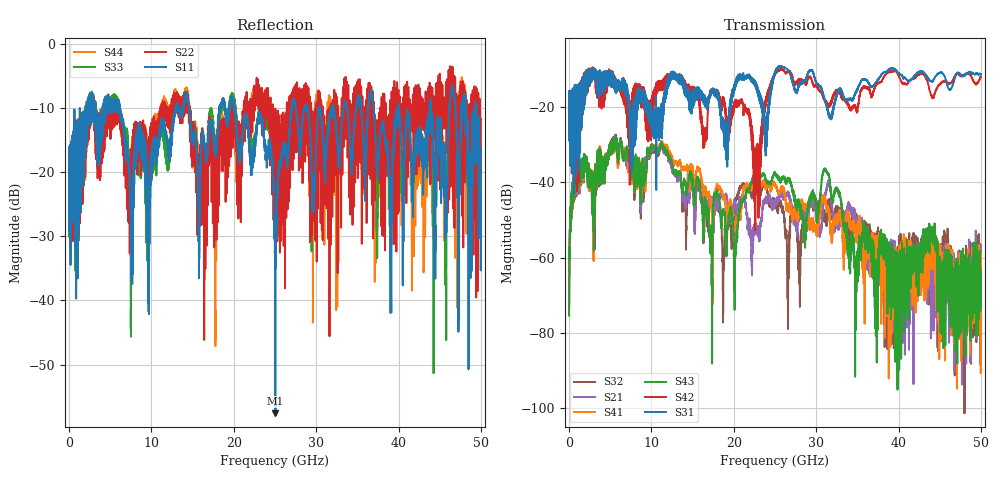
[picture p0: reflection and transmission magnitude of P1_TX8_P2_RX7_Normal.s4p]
!Keysight Technologies,N5225B,MY57041031,A.13.20.10
!Date: Friday, May 31, 2019 11:39:04
!Correction: S11(Full 4 Port(1,2,3,4))
!S12(Full 4 Port(1,2,3,4))
!S13(Full 4 Port(1,2,3,4))
!S14(Full 4 Port(1,2,3,4))
!S21(Full 4 Port(1,2,3,4))
!S22(Full 4 Port(1,2,3,4))
!S23(Full 4 Port(1,2,3,4))
!S24(Full 4 Port(1,2,3,4))
!S31(Full 4 Port(1,2,3,4))
!S32(Full 4 Port(1,2,3,4))
!S33(Full 4 Port(1,2,3,4))
!S34(Full 4 Port(1,2,3,4))
!S41(Full 4 Port(1,2,3,4))
!S42(Full 4 Port(1,2,3,4))
!S43(Full 4 Port(1,2,3,4))
!S44(Full 4 Port(1,2,3,4))
!S4P File: Measurements: <S11,S12,S13,S14>,
!<S21,S22,S23,S24>,
!<S31,S32,S33,S34>,
!<S41,S42,S43,S44>:
# Hz S  dB  R 50.0
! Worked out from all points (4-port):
!   5000 points, 10 MHz to 50 GHz, reference 50 ohm
!   strongest paths, dB at 10 MHz, 12.51 GHz, 25.01 GHz, 37.51 GHz, 50 GHz:
!     S31: -19.6, -10.7, -11.1, -12.7, -11.3
!     S42: -19.3, -12.1, -11.4, -13.7, -12.0
!     S43: -75.4, -35.1, -37.6, -66.2, -70.9
!     S41: -65.5, -33.4, -40.2, -55.2, -60.5
!     S21: -62.9, -36.6, -44.9, -58.5, -62.3
!     S32: -63.7, -36.4, -45.9, -56.3, -66.4
!   lowest |S11| = -57.6 dB at 25.05 GHz (marker M1), VSWR 1.00, Z = 49.9 - j0.0463 ohm
!   |S11| at or under -10 dB: 6.186 GHz to 12.89 GHz (6.703 GHz wide, 70.3 % of centre); 20.1 GHz to 26.99 GHz (6.891 GHz wide, 29.3 % of centre); 40 GHz to 43.77 GHz (3.763 GHz wide, 8.98 % of centre)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
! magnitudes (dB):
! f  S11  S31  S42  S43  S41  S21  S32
! 10 MHz  -19.5  -19.6  -19.3  -75.4  -65.5  -62.9  -63.7
! 820 MHz  -18.8  -18.2  -17.2  -36.5  -36.5  -36.8  -37.2
! 5.5 GHz  -8.4  -12.1  -13.8  -28.8  -29.0  -28.4  -28.0
! 20.19 GHz  -10.7  -14.7  -19.6  -58.9  -54.3  -45.7  -44.4
! 22.8 GHz  -12.6  -14.2  -37.2  -38.7  -40.8  -53.3  -42.7
! 25.05 GHz  -57.6  -10.5  -11.3  -37.6  -40.6  -44.4  -46.1
! 50 GHz  -22.5  -11.3  -12.0  -70.9  -60.5  -62.3  -66.4
